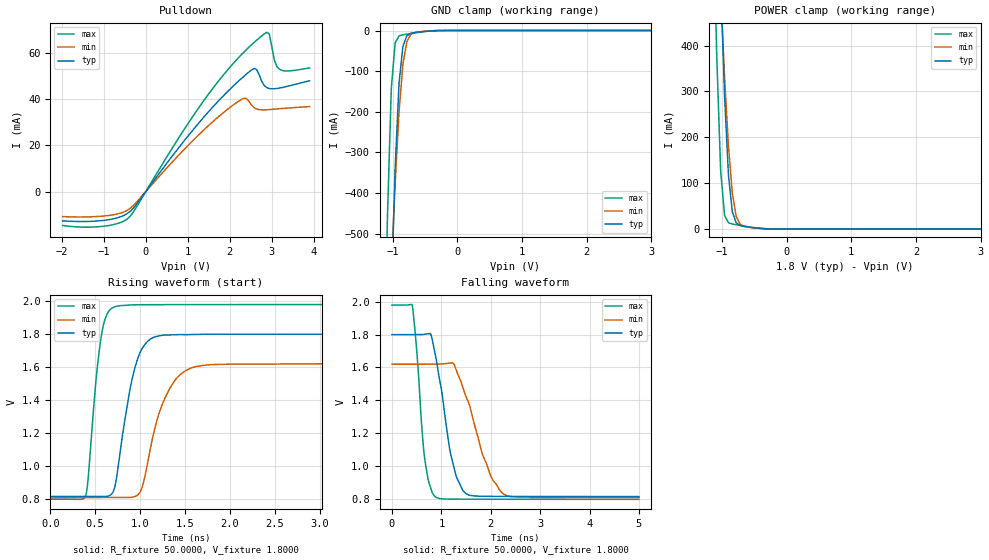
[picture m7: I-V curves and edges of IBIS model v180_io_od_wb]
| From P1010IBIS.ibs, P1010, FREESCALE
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[Model] v180_io_od_wb
|   Model v180_io_od_wb
| This model has derived from v180_wb
| Only applicable curves and parameters are copied
Model_type I/O_open_drain
Polarity   Non-Inverting
Enable   Active-High
Vinl =   0.5400V
Vinh =   1.2600V
Vmeas =  0.9000V
Cref =   0.0F
Rref =   50.0000
Vref =   0.9000V
C_comp   2.1221pF   1.9600pF   2.4667pF
[Temperature Range]   85.0000   0.1250k   -40.0000
[Voltage Range]   1.8000V   1.6200V   1.9800V
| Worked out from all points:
|   slope of the pulldown table from 0 to 0.27 V, typ, clamps not added: 40.4 ohm
|   GND clamp passes 1 mA (typ) near -0.40 V on its own axis
|   POWER clamp passes 1 mA (typ) near -0.37 V on its own axis
|   rising waveform, R_fixture 50.0000, V_fixture 1.8000: 20-80 % time 186ps typ, 252ps min, 118ps max; typ from 0.814 V to 1.8 V
|   falling waveform, R_fixture 50.0000, V_fixture 1.8000: 20-80 % time 320ps typ, 504ps min, 177ps max; typ from 1.8 V to 0.814 V
[Pulldown]
|Voltage   I(typ)   I(min)   I(max)
-1.98V    -12.66mA   -10.83mA   -14.68mA
-1.02V    -12.5mA    -10.6mA    -15.04mA
-420mV    -9.259mA   -7.874mA   -11.53mA
1.2V      28.39mA    23.53mA    34.72mA
2.22V     48.08mA    39.31mA    58.26mA
2.4V      50.97mA    40.32mA    61.59mA
2.58V     53.33mA    36.41mA    64.65mA
2.88V     45.1mA     35.47mA    69.04mA
2.94V     44.69mA    35.54mA    68.34mA
3.06V     44.58mA    35.73mA    57.1mA
3.18V     44.88mA    35.91mA    53.1mA
3.9V      48.03mA    36.86mA    53.61mA
[GND_clamp]
|Voltage   I(typ)   I(min)   I(max)
-1.98V    -8.37A     -5.087A    -9.647A
-1.14V    -1.459A    -1.082A    -930.9mA
-1.08V    -1.036A    -828.3mA   -462.6mA
-1.02V    -653.4mA   -590.2mA   -143.2mA
-960mV    -338mA     -376mA     -30.24mA
-900mV    -129.6mA   -200.5mA   -13.2mA
-840mV    -38.64mA   -82.98mA   -10.47mA
-780mV    -13.16mA   -27.75mA   -8.896mA
-720mV    -7.156mA   -9.942mA   -7.424mA
-660mV    -5.182mA   -5.042mA   -5.995mA
-240mV    -56.29uA   -39.98uA   -23.22uA
3.9V      0A         0A         0A
[POWER_clamp]
|Voltage   I(typ)   I(min)   I(max)
-1.92V    6.087A     4.039A     6.601A
-1.14V    1.168A     928.8mA    722.7mA
-1.08V    840.5mA    715.6mA    374.8mA
-1.02V    542mA      514.8mA    127.3mA
-960mV    291.6mA    333.1mA    29.94mA
-900mV    119mA      182.4mA    13.62mA
-840mV    37.87mA    78.7mA     10.87mA
-780mV    13.54mA    27.69mA    9.257mA
-720mV    7.641mA    10.53mA    7.748mA
-660mV    5.688mA    5.717mA    6.285mA
-240mV    130.6uA    144.5uA    23.85uA
3.96V     0A         0A         0A
[Ramp]
| variable   typ   min   max
dV/dt_r  0.5852/0.3523n   0.4766/0.5910n   0.7103/0.1825n
dV/dt_f  0.5912/0.3203n   0.4869/0.5037n   0.7093/0.1774n
R_load = 50.0000
[Rising Waveform]
R_fixture= 50.0000
V_fixture= 1.8000
V_fixture_min= 1.6200
V_fixture_max= 1.9800
|time   V(typ)   V(min)   V(max)
0s        814.3mV    807.8mV    797.5mV
396ps     814.4mV    807.8mV    822.5mV
562.2ps   814.6mV    807.9mV    1.767V
703.9ps   847.6mV    808.1mV    1.962V
937.1ps   1.584V     812.5mV    1.978V
1.029ns   1.718V     879.5mV    1.978V
1.15ns    1.78V      1.194V     1.979V
1.353ns   1.795V     1.491V     1.979V
1.633ns   1.798V     1.604V     1.979V
5ns       1.8V       1.62V      1.98V
[Falling Waveform]
R_fixture= 50.0000
V_fixture= 1.8000
V_fixture_min= 1.6200
V_fixture_max= 1.9800
|time   V(typ)   V(min)   V(max)
0s        1.8V       1.62V      1.98V
412.1ps   1.8V       1.62V      1.974V
653.6ps   1.802V     1.62V      1.066V
782.7ps   1.803V     1.62V      866.8mV
876.4ps   1.681V     1.62V      813.2mV
1.188ns   1.073V     1.628V     798.8mV
1.495ns   832.9mV    1.426V     798.3mV
1.981ns   815.8mV    953.9mV    797.9mV
2.294ns   815.3mV    824.2mV    797.7mV
5ns       814.5mV    808.3mV    797.6mV
